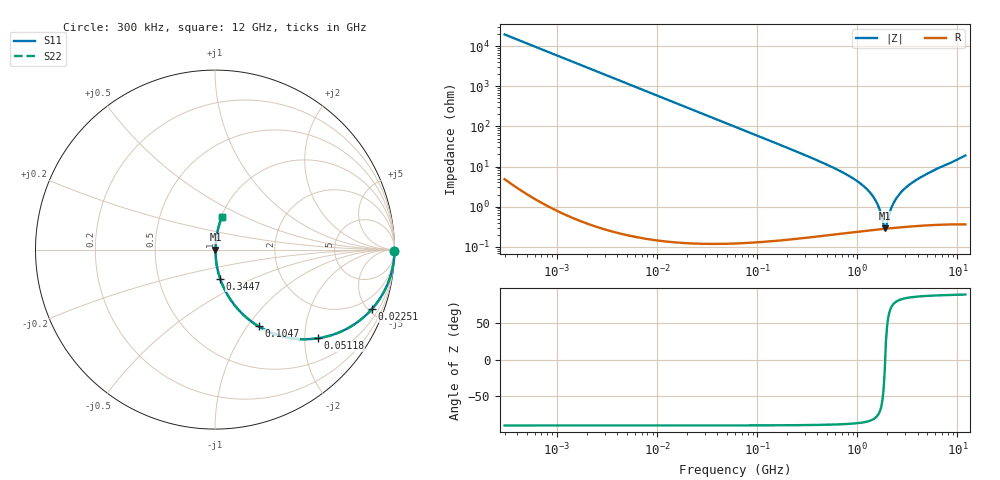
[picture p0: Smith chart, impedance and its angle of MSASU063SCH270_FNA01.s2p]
! MSASU063SCH270_FNA01  S-PARAMETER MODEL  ( General Type )
! Model Generated by TAIYO YUDEN Corporation (http://www.ty-top.com)
! Version 4.0
! TAIYO YUDEN Control No. 120810
! Copyright(c) 2009 TAIYO YUDEN CO.,LTD. All Rights Reserved.
! Product Description (link to TY-COMPAS)
! https://ds.yuden.co.jp/TYCOMPAS/or/detail?pn=MSASU063SCH270JFNA01&u=M
! Products Name : Multilayer Ceramic Capacitors
! Characteristics :
!  Capacitance : 27 pF , Rated Voltage : 50V , TCC : CH / C0H
!  Case Size : 0.6 x 0.3 / 0.024 x 0.012 [mm/inch] , Thickness : 0.3 / 0.012 [mm/inch]
!  (Conditions: Temperature = 25 degC , DC Bias Current/Voltage = 0A / 0V)
! External Node Assignments :
!  1  o---| |---o  2
! GND o---------o GND
! Frequency Range : 0.3MHz  -  12000MHz  [ 401 STEP ]
# MHz S RI R 50
! Freq[MHz].  S11 Real  S11 Imag  S21 Real  S21 Imag  S12 Real  S12 Imag  S22 Real  S22 Imag
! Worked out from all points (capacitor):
!   401 points, 300 kHz to 12 GHz, reference 50 ohm
!   read as one part in series: C = 26.8 pF near 316.3 kHz
!   lowest |Z| = 288 mohm at 1.879 GHz (marker M1)
!   series resonance near 1.897 GHz, so ESL is about 260 pH
!   S11 on the Smith chart (normalised r, x): 300 kHz: open; 22.51 MHz: 1.00, -5.27; 51.18 MHz: 1.00, -2.32; 104.7 MHz: 1.00, -1.13; 344.7 MHz: 1.00, -0.33; 12 GHz: 1.01, +0.38
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0.3  1 -0.00505  2.68e-05 0.00505  2.68e-05 0.00505  1 -0.00505
1.769972  0.9991 -0.0298  0.000892 0.0298  0.000892 0.0298  0.9991 -0.0298
10.44266  0.9699 -0.1706  0.0301 0.1706  0.0301 0.1706  0.9699 -0.1706
22.51442  0.8741 -0.3315  0.1259 0.3315  0.1259 0.3315  0.8741 -0.3315
51.18236  0.5732 -0.4941  0.4268 0.4941  0.4268 0.4941  0.5732 -0.4941
60  0.4942 -0.4994  0.5058 0.4994  0.5058 0.4994  0.4942 -0.4994
104.6549  0.2428 -0.4277  0.7572 0.4277  0.7572 0.4277  0.2428 -0.4277
177.7716  0.0998 -0.2976  0.9002 0.2976  0.9002 0.2976  0.0998 -0.2976
344.7396  0.0286 -0.1615  0.9714 0.1615  0.9714 0.1615  0.0286 -0.1615
353.9943  0.0271 -0.1572  0.9729 0.1572  0.9729 0.1572  0.0271 -0.1572
763.2128  0.00637 -0.0647  0.9936 0.0647  0.9936 0.0647  0.00637 -0.0647
1197.383  0.00335 -0.0297  0.9967 0.0297  0.9967 0.0297  0.00335 -0.0297
1519.776  0.00283 -0.014  0.9972 0.014  0.9972 0.014  0.00283 -0.014
1829.429  0.00277 -0.00233  0.9972 0.00233  0.9972 0.00233  0.00277 -0.00233
1878.541  0.00278 -0.000714  0.9972 0.000714  0.9972 0.000714  0.00278 -0.000714
1980.756  0.00282 0.00279  0.9972 -0.00279  0.9972 -0.00279  0.00282 0.00279
2088.533  0.00289 0.00598  0.9971 -0.00598  0.9971 -0.00598  0.00289 0.00598
2261.293  0.00303 0.0108  0.997 -0.0108  0.997 -0.0108  0.00303 0.0108
2448.343  0.00321 0.0157  0.9968 -0.0157  0.9968 -0.0157  0.00321 0.0157
3276.641  0.00433 0.0342  0.9957 -0.0342  0.9957 -0.0342  0.00433 0.0342
5278.635  0.00841 0.0704  0.9916 -0.0704  0.9916 -0.0704  0.00841 0.0704
12000  0.0376 0.1809  0.9624 -0.1809  0.9624 -0.1809  0.0376 0.1809
